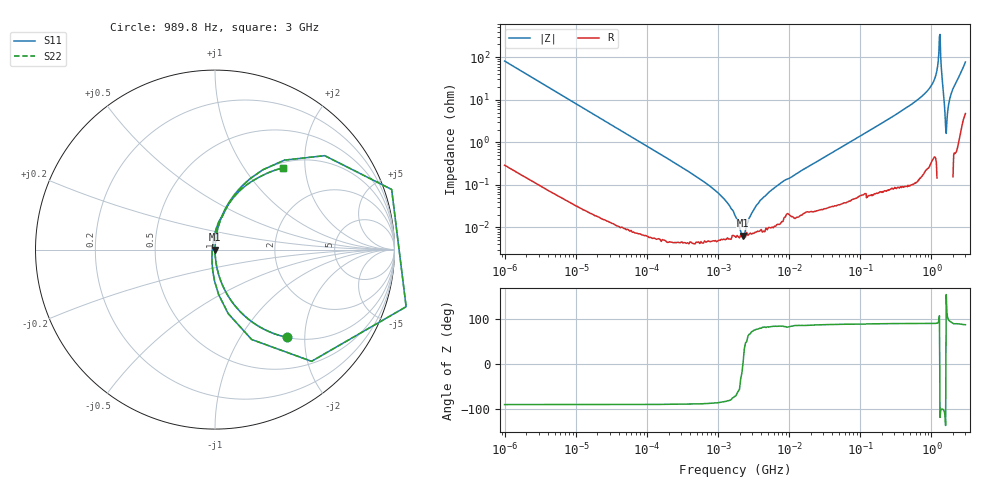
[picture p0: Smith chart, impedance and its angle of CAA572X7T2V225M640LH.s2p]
! S-Parameter Data Generated by TDK Corporation
! Copyright(C) 2020 TDK Corporation.
! All Rights Reserved.
! TDK P/N: CAA572X7T2V225M640LH (Multilayer Ceramic Chip Capacitor)
! Property: C=2.2uF
! Size(LxWxT): 6x5x6.4mm
! Model Type: s2p (Touchstone File Format Version 1.0)
! Frequency: DC=Yes Start=0.000989846MHz Stop=3000MHz 463points Log-sweep
! Model Generated on Nov. 18, 2020
! Port Assignments:
!  1 ---| |--- 2
! Applicable Conditions:
!  Temperature = 25 degC
!  DC Bias Voltage = 0 V
!  Small Signal Operation
! Terms and conditions regarding TDK Simulation Models
! (1)This simulation model is being provided solely for informational purposes. Please refer to the specifications of the products in terms of detailed characteristics of such products.
! (2)In no event shall TDK Corporation of any of its subsidiaries be liable for any loss or damage arising, directly or indirectly,
!  From any information contained in this simulation model, including, but not limited to loss or damages arising from any inaccuracies, omissions or errors in connection with such information.
! (3)Any and all copyrights on this simulation model are owned by TDK Corporation.
!  Duplication or redistribution of this simulation model without prior written permission from TDK Corporation is prohibited.
! (4)This simulation model is subject to any modification or change without any prior notice.
! (5)Neither TDK Corporation nor any of its subsidiaries shall make any warranty, express or implied,
!  Including but not limited to the correctness, implied warranties of merchantability and fitness for a particular purpose with respect to this simulation models.
! (6)The use of this simulation model shall be deemed to have consented to the terms and conditions hereof.
# Hz S MA R 50
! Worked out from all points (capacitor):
!   462 points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, 989.8 Hz to 3 GHz, reference 50 ohm
!   read as one part in series: C = 1.98 uF near 1.07 kHz
!   lowest |Z| = 6.42 mohm at 2.243 MHz (marker M1)
!   series resonance near 2.228 MHz, so ESL is about 2.6 nH
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989.846  0.6298 -50.8  0.7745 39.0  0.7745 39.0  0.6298 -50.8
2625.441  0.2934 -72.7  0.9549 17.1  0.9549 17.1  0.2934 -72.7
12024.64  0.06719 -85.9  0.9975 3.9  0.9975 3.9  0.06719 -85.9
146075.1  0.005552 -89.1  0.9999 0.3  0.9999 0.3  0.005552 -89.1
914132.1  0.0007341 -86.1  1 0.0  1 0.0  0.0007341 -86.1
1774518  0.0001746 -70.3  0.9999 0.0  0.9999 0.0  0.0001746 -70.3
2242604  6.418e-05 4.1  0.9999 -0.0  0.9999 -0.0  6.418e-05 4.1
5291161  0.0006971 81.7  0.9999 -0.0  0.9999 -0.0  0.0006971 81.7
2.073191e7  0.003005 85.3  0.9998 -0.2  0.9998 -0.2  0.003005 85.3
2.507343e8  0.03546 86.7  0.9986 -2.0  0.9986 -2.0  0.03546 86.7
6.821091e8  0.1085 83.0  0.9927 -6.2  0.9927 -6.2  0.1085 83.0
1.059487e9  0.2507 74.6  0.9641 -14.5  0.9641 -14.5  0.2507 74.6
1.171007e9  0.3873 66.8  0.9189 -22.8  0.9189 -22.8  0.3873 66.8
1.243477e9  0.6312 52.2  0.79 -39.1  0.79 -39.1  0.6312 52.2
1.294266e9  1.04 18.8  0.3355 -87.3  0.3355 -87.3  1.04 18.8
1.374365e9  0.5409 -67.8  0.9403 32.2  0.9403 32.2  0.5409 -67.8
1.430499e9  0.2518 -85.3  1.011 14.4  1.011 14.4  0.2518 -85.3
1.54974e9  0.04757 -111.0  1.018 2.5  1.018 2.5  0.04757 -111.0
1.613037e9  0.01645 152.6  1.015 -0.4  1.015 -0.4  0.01645 152.6
1.782824e9  0.09523 89.6  1.004 -5.4  1.004 -5.4  0.09523 89.6
1.931433e9  0.1518 82.6  0.992 -8.7  0.992 -8.7  0.1518 82.6
3e9  0.5933 50.2  0.7693 -36.3  0.7693 -36.3  0.5933 50.2
